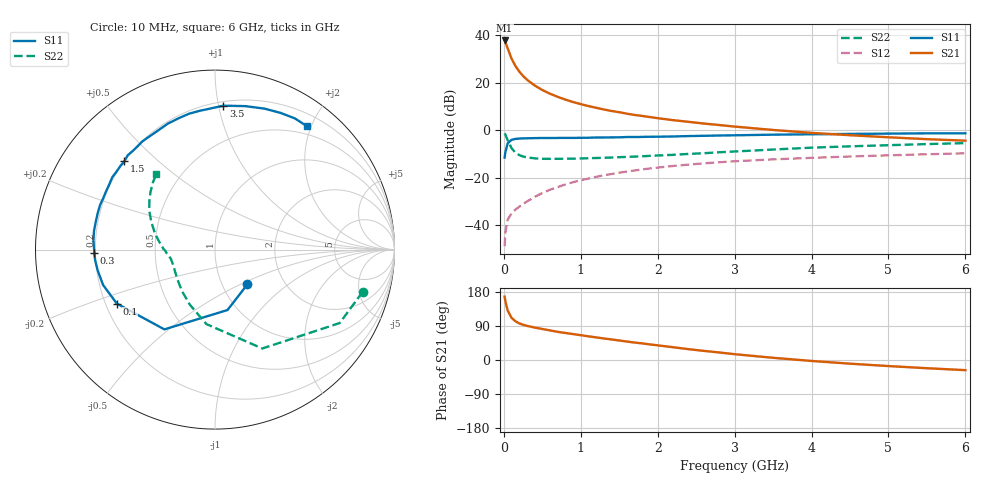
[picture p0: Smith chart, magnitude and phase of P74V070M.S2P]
! SIEMENS Small Signal Semiconductors
! BFP196
! Si NPN RF Bipolar Junction Transistor in SOT143
! VCE = 4 V  IC = 70 mA
! Common Emitter S-Parameters:  May  1996
# GHz  S  MA  R  50
!  f  S11  S21  S12  S22
! GHz  MAG  ANG  MAG  ANG  MAG  ANG  MAG  ANG
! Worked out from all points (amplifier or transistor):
!   36 points, 10 MHz to 6 GHz, reference 50 ohm
!   highest |S21| = 37.8 dB at 10 MHz (marker M1)
!   |S21| within 3 dB of that: start of sweep to 46.1 MHz
!   unconditionally stable (mu >= 1): 405.8 MHz to 4.453 GHz
!   at 250 MHz: K = 0.88, MSG = 26.9 dB, |S12| = -31.1 dB
!   at 1.4 GHz: K = 1.09, MAG = 11.5 dB, |S12| = -18.5 dB
!   at 6 GHz: K = 0.98, MSG = 2.7 dB, |S12| = -9.8 dB
!   S11 on the Smith chart (normalised r, x): 10 MHz: 1.31, -0.55; 100 MHz: 0.25, -0.24; 300 MHz: 0.20, -0.01; 1.5 GHz: 0.20, +0.39; 3.5 GHz: 0.23, +1.03; 6 GHz: 0.37, +1.94
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0.01  0.2649 -47.2  77.34 167.2  0.0036 75.6  0.8557 -16.0
0.02  0.3438 -78.3  71.38 154.9  0.007 72.0  0.8062 -30.5
0.05  0.5264 -122.4  52.62 130.5  0.0131 56.0  0.6109 -64.4
0.1  0.6243 -151.2  32.15 111.3  0.0176 49.7  0.4177 -96.6
0.15  0.6541 -162.5  22.49 102.3  0.0212 51.5  0.3364 -114.9
0.2  0.664 -170.0  17.19 96.7  0.0243 54.9  0.2988 -126.9
0.25  0.6705 -175.0  13.8 92.9  0.028 56.9  0.2775 -135.8
0.3  0.6726 -178.5  11.57 90.1  0.0314 60.3  0.2666 -141.7
0.4  0.6792 175.6  8.745 85.7  0.0393 61.8  0.2547 -150.6
0.5  0.6821 171.2  6.995 81.8  0.0472 63.9  0.2494 -156.2
0.6  0.6822 166.5  5.843 78.1  0.0556 64.5  0.2484 -160.2
0.7  0.6844 162.4  5.021 74.3  0.0633 64.3  0.2487 -163.1
0.8  0.6868 158.7  4.393 71.4  0.0718 63.6  0.2499 -165.4
0.9  0.6854 155.4  3.909 68.4  0.0801 62.7  0.2505 -167.6
1.1  0.6919 148.5  3.214 62.4  0.0957 61.0  0.2561 -170.6
1.5  0.7048 135.7  2.386 51.5  0.1268 56.0  0.269 -175.6
2.2  0.7348 115.9  1.621 33.7  0.1758 45.4  0.302 175.0
3  0.7776 96.5  1.187 15.3  0.2209 33.4  0.3545 163.0
3.5  0.8031 86.7  1.008 5.8  0.2424 26.4  0.3905 155.8
4.5  0.8323 70.7  0.781 -9.7  0.2787 14.3  0.4559 143.3
5.5  0.8557 58.7  0.645 -21.7  0.3103 3.6  0.5084 133.0
6  0.8575 53.3  0.6 -26.8  0.3249 -2.1  0.5325 128.1
